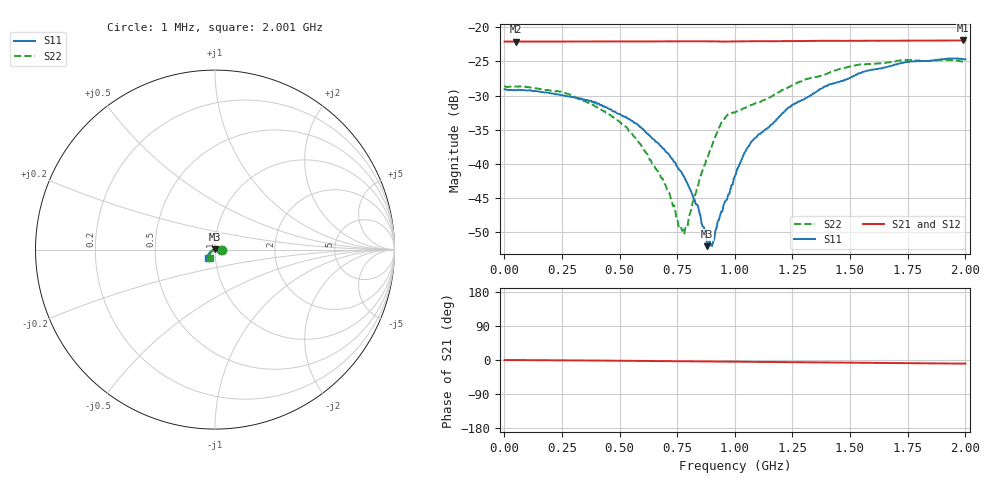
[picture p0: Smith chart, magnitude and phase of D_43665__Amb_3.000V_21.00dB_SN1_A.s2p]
! device id: 43665_
! dir: \\malibu\benchdata\1_engineers\tn_data\43665_75ohm\new\sparar\43665_\amb\3p000v\21p00db
! Serial: 1
! Insertion: A
! Temp: Amb
! VDD: 3.000V
! Attenuation Step: 21.00dB
! IDD: 1.447470e+00mA
! FILE NAME
! DATE 03-27-2009 08:38:30
! CORRECTED  DATA
#  Hz  S  RI  R  75
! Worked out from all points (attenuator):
!   401 points, 1 MHz to 2.001 GHz, reference 75 ohm
!   highest |S21| = -21.95 dB at 1.991 GHz (marker M1); lowest = -22.1 dB at 51 MHz (marker M2)
!   lowest |S11| = -52.0 dB at 881 MHz (marker M3), VSWR 1.01, Z = 74.9 + j0.37 ohm
!   |S11| at or under -10 dB: start of sweep to end of sweep
!   |S22| runs from -50.3 to -24.8 dB; largest |S21 - S12| = 0.00038
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1000000  0.0352 -0.000231  0.0784 -0.000123  0.0786 -7.98e-05  0.0372 -0.000287
5.1e7  0.0345 0.000945  0.0784 -0.000253  0.0785 -0.000246  0.0368 0.00145
3.36e8  0.0297 0.00516  0.0785 -0.00174  0.0786 -0.00163  0.0273 0.0104
5.26e8  0.0212 0.00665  0.0786 -0.00287  0.0787 -0.00278  0.0161 0.00959
6.71e8  0.0127 0.0059  0.0786 -0.00368  0.0786 -0.00357  0.00578 0.00635
7.16e8  0.0102 0.0056  0.0786 -0.00399  0.0787 -0.00384  0.00294 0.00541
7.61e8  0.00762 0.0048  0.0787 -0.00435  0.0787 -0.00418  -0.000903 0.00345
7.81e8  0.00657 0.0046  0.0787 -0.00449  0.0787 -0.00435  -0.00233 0.00198
8.41e8  0.00279 0.00403  0.0787 -0.005  0.0787 -0.00482  -0.00652 -0.0025
8.81e8  -0.000439 0.00247  0.0786 -0.00539  0.0787 -0.00518  -0.00917 -0.00593
8.91e8  -0.00113 0.00249  0.0786 -0.00545  0.0786 -0.00525  -0.0102 -0.00698
9.06e8  -0.00224 0.00152  0.0785 -0.00558  0.0786 -0.00538  -0.0118 -0.00823
9.51e8  -0.00498 0.00022  0.0783 -0.0057  0.0783 -0.0055  -0.0185 -0.0102
1.001e9  -0.00814 -0.000438  0.0785 -0.00567  0.0785 -0.00551  -0.022 -0.00891
1.046e9  -0.0122 -0.00195  0.0787 -0.0061  0.0788 -0.00586  -0.023 -0.0115
1.081e9  -0.0146 -0.00374  0.0787 -0.00654  0.0788 -0.00633  -0.0236 -0.0139
1.231e9  -0.0238 -0.0099  0.0787 -0.00755  0.0789 -0.00729  -0.0274 -0.0239
1.336e9  -0.0286 -0.0152  0.0789 -0.00825  0.0791 -0.00803  -0.03 -0.0303
1.546e9  -0.0375 -0.027  0.0788 -0.0101  0.0791 -0.00989  -0.0325 -0.0424
1.671e9  -0.0396 -0.0332  0.0788 -0.0109  0.079 -0.0109  -0.0319 -0.0452
1.991e9  -0.0377 -0.0446  0.0788 -0.0132  0.079 -0.0133  -0.0276 -0.0487
2.001e9  -0.0374 -0.0446  0.0788 -0.0132  0.0789 -0.0133  -0.0274 -0.0484
